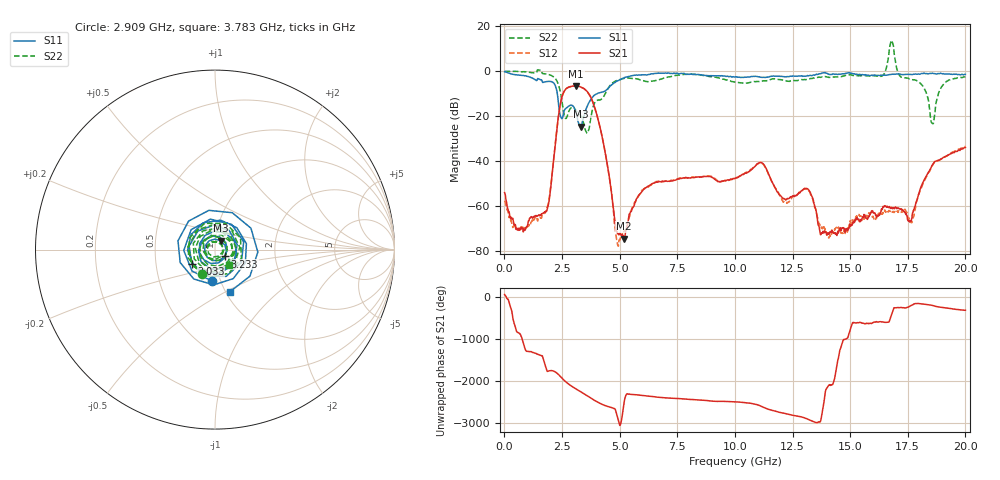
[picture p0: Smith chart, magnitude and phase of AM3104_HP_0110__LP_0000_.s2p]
!Created with skrf (http://scikit-rf.org).
# Hz S RI R 50.0
!freq ReS11 ImS11 ReS21 ImS21 ReS12 ImS12 ReS22 ImS22
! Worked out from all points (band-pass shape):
!   1601 points, 10 MHz to 20 GHz, reference 50 ohm
!   highest |S21| = -6.55 dB at 3.108 GHz (marker M1); lowest = -74.4 dB at 5.182 GHz (marker M2)
!   |S21| within 3 dB of the highest: 2.564 GHz to 3.63 GHz (1.067 GHz wide, 34.4 % of centre)
!   lowest |S11| = -24.6 dB at 3.333 GHz (marker M3), VSWR 1.12, Z = 53 + j5.23 ohm
!   |S11| at or under -10 dB: 2.296 GHz to 4.023 GHz (1.727 GHz wide, 54.7 % of centre)
!   |S22| runs from -27.6 to 13.7 dB; largest |S21 - S12| = 0.026
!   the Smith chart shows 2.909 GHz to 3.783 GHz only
!   S11 on the Smith chart (normalised r, x): 2.909 GHz: 0.91, -0.33; 3.033 GHz: 0.76, -0.12; 3.233 GHz: 1.11, -0.09; 3.783 GHz: 1.04, -0.53
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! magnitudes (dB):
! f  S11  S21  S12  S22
! 10 MHz  -0.2  -54.0  -57.6  -0.1
! 597.2 MHz  -1.7  -70.0  -70.0  -0.1
! 1.797 GHz  -4.6  -62.4  -62.0  -1.2
! 2.446 GHz  -20.4  -13.6  -13.7  -10.1
! 2.909 GHz  -15.1  -6.8  -6.8  -16.1
! 3.033 GHz  -16.4  -6.6  -6.6  -16.4
! 3.108 GHz  -18.3  -6.5  -6.5  -17.7
! 3.233 GHz  -23.5  -6.7  -6.8  -19.2
! 3.333 GHz  -24.6  -7.1  -7.2  -20.1
! 3.346 GHz  -24.4  -7.1  -7.2  -20.5
! 3.783 GHz  -12.1  -12.4  -12.4  -18.8
! 4.87 GHz  -4.5  -71.2  -74.9  -4.2
! 5.182 GHz  -2.9  -74.4  -71.1  -3.2
! 6.682 GHz  -0.9  -49.2  -48.9  -3.9
! 10.01 GHz  -2.6  -47.7  -47.7  -4.8
! 11.14 GHz  -2.7  -40.6  -40.8  -4.4
! 13.34 GHz  -2.0  -55.7  -56.0  -3.2
! 14.08 GHz  -1.4  -72.5  -74.1  -2.8
! 16.68 GHz  -1.5  -60.5  -62.1  7.2
! 17.59 GHz  -1.5  -67.1  -66.5  -3.5
! 18.56 GHz  -0.9  -41.7  -41.9  -23.2
! 20 GHz  -1.4  -33.9  -33.4  -2.5
